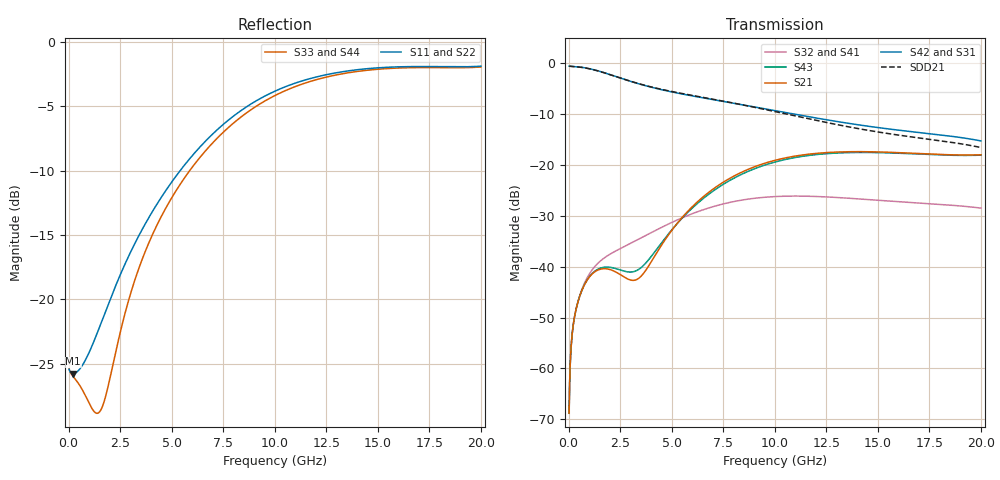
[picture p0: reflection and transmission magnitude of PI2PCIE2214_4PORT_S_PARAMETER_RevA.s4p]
! NPort=4 DATA=800 NOISE=0 GROUPDELAY=0 COMPLEX_DATAFORMAT=POLAR
! NumOfBlock=1 NumOfParam=0
! .MODEL Smodel S TSTONEFILE=PI2PCIE2214_4PORT_S_PARAMETER_RevA.s4p TYPE=S
!  -- The above .MODEL line can be used for the S element in the netlist.
! PORT DEFINITION
! PORT1 = INPUT+
! PORT2 = INPUT-
! PORT3 = OUTPUT+
! PORT4 = OUTPUT-
# Hz S MA R  50
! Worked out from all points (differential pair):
!   800 points, 25 MHz to 20 GHz, reference 50 ohm
!   strongest paths, dB at 25 MHz, 5.025 GHz, 10.03 GHz, 15.03 GHz, 20 GHz:
!     S42: -0.5, -5.6, -9.3, -12.6, -15.2
!     S31: -0.5, -5.6, -9.3, -12.6, -15.2
!     S21: -68.8, -32.7, -19.0, -17.4, -18.0
!     S43: -68.8, -32.6, -19.4, -17.5, -18.0
!     S32: -68.8, -31.2, -26.2, -26.9, -28.5
!     S41: -68.8, -31.2, -26.2, -26.9, -28.5
!   taken as a pair (ports 2,1 in; 4,3 out), SDD21 dB: -0.5, -5.5, -9.5, -13.5, -16.6
!   lowest |S11| = -25.8 dB at 225 MHz (marker M1), VSWR 1.11, Z = 54.8 - j2.37 ohm
!   |S11| at or under -10 dB: start of sweep to 5.411 GHz
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2.5e7  0.05348 -4.2  0.0003628 86.7  0.94 -0.7  0.0003614 86.6
       0.0003628 86.7  0.05348 -4.2  0.0003614 86.6  0.94 -0.7
       0.94 -0.7  0.0003614 86.6  0.05354 -3.3  0.0003629 86.7
       0.0003614 86.6  0.94 -0.7  0.0003629 86.7  0.05354 -3.3
2.25e8  0.05138 -24.8  0.002679 70.4  0.9343 -5.7  0.002676 70.2
        0.002679 70.4  0.05137 -24.8  0.002676 70.2  0.9343 -5.7
        0.9343 -5.7  0.002676 70.2  0.05001 -16.7  0.002677 70.8
        0.002676 70.2  0.9343 -5.7  0.002677 70.8  0.05001 -16.6
1.725e9  0.08687 -157.3  0.009569 46.7  0.8107 -40.0  0.01219 43.4
         0.009568 46.7  0.0867 -157.3  0.01219 43.4  0.8108 -40.0
         0.8108 -40.0  0.01219 43.4  0.04006 -157.1  0.009885 50.2
         0.01219 43.4  0.8108 -40.0  0.009884 50.2  0.03992 -157.1
3.375e9  0.1746 114.9  0.007625 83.4  0.6325 -66.7  0.01856 28.4
         0.007626 83.4  0.1744 114.8  0.01856 28.4  0.6327 -66.7
         0.6326 -66.7  0.01856 28.4  0.1297 98.9  0.009346 80.6
         0.01856 28.4  0.6327 -66.7  0.009346 80.6  0.1295 98.8
8.7e9  0.5644 -10.3  0.09066 86.0  0.3831 -129.9  0.04623 -45.1
       0.09066 86.0  0.5643 -10.3  0.04623 -45.1  0.3832 -129.9
       0.3832 -129.9  0.04624 -45.1  0.5351 -13.1  0.08661 84.3
       0.04624 -45.1  0.3833 -129.9  0.08662 84.3  0.535 -13.1
1.365e10  0.7739 -66.3  0.1354 34.1  0.2561 176.9  0.0471 -122.7
          0.1354 34.1  0.7739 -66.3  0.0471 -122.7  0.2561 176.9
          0.2561 177.0  0.04712 -122.7  0.7612 -66.9  0.1328 34.3
          0.04712 -122.7  0.2562 176.9  0.1328 34.3  0.7611 -66.9
2e10  0.8055 -97.8  0.1262 5.3  0.1728 100.9  0.03772 146.2
      0.1262 5.3  0.8054 -97.8  0.03772 146.2  0.1728 100.9
      0.1729 101.0  0.03773 146.2  0.7993 -97.9  0.1252 5.7
      0.03773 146.2  0.1729 101.0  0.1252 5.7  0.7992 -97.9
